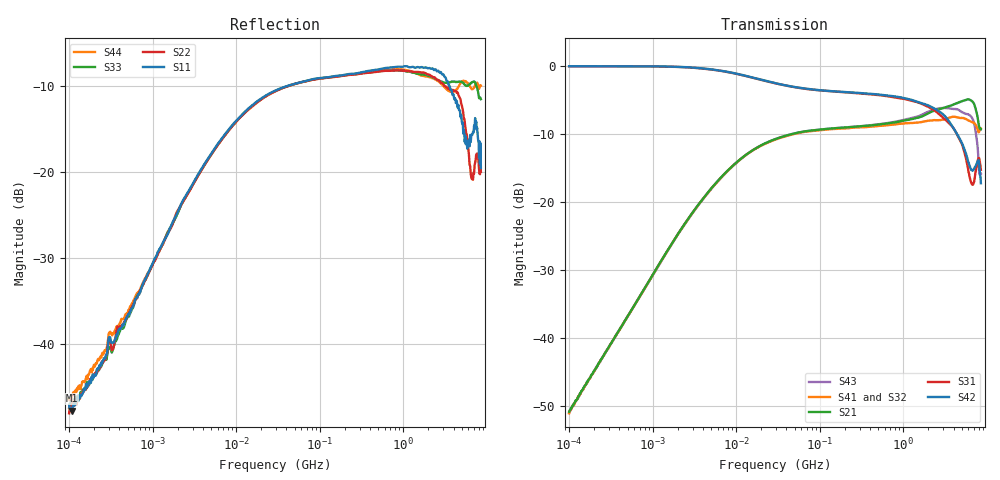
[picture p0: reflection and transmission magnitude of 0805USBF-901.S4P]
# Hz S dB R 50
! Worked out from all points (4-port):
!   801 points, 100 kHz to 8.5 GHz, reference 50 ohm
!   strongest paths, dB at 100 kHz, 1.721 MHz, 29.51 MHz, 502.3 MHz, 8.5 GHz:
!     S42: 0.0, -0.1, -2.5, -4.2, -17.2
!     S31: 0.0, -0.1, -2.5, -4.3, -15.3
!     S21: -50.9, -26.0, -10.7, -8.6, -9.3
!     S41: -51.1, -26.0, -10.8, -8.8, -9.2
!     S32: -51.0, -26.1, -10.8, -8.9, -8.9
!     S43: -51.1, -26.1, -10.7, -8.6, -15.8
!   lowest |S11| = -47.7 dB at 108.3 kHz (marker M1), VSWR 1.01, Z = 50.1 + j0.395 ohm
!   |S11| at or under -10 dB: start of sweep to 39.97 MHz; 3.593 GHz to end of sweep
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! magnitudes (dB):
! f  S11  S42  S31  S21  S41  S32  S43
! 100 kHz  -47.1  0.0  0.0  -50.9  -51.1  -51.0  -51.1
! 108.3 kHz  -47.7  0.0  0.0  -50.1  -50.2  -50.3  -50.2
! 24.59 MHz  -10.9  -2.3  -2.3  -11.1  -11.2  -11.2  -11.1
! 1.824 GHz  -7.8  -5.6  -5.8  -7.2  -8.1  -8.2  -6.9
! 4.564 GHz  -12.2  -10.3  -10.5  -5.4  -7.6  -8.2  -6.4
! 6.428 GHz  -16.5  -15.1  -17.0  -5.0  -8.2  -8.2  -7.4
! 8.5 GHz  -19.5  -17.2  -15.3  -9.3  -9.2  -8.9  -15.8
